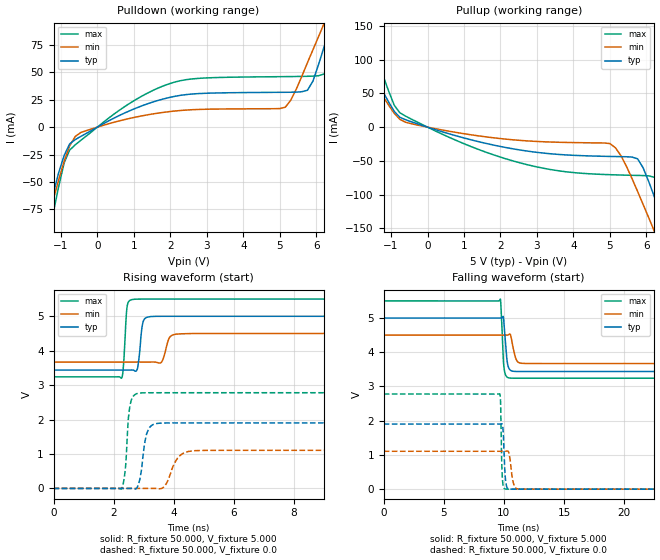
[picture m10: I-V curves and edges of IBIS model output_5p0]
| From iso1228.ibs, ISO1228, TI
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|   Model output_5p0
[Model] output_5p0
Model_type Output
Polarity   Non-Inverting
Enable   Active-High
Vmeas = 2.5
Vref = 0
Cref = 15pF
Rref = 1000
C_comp   0.978pF   1.050pF   0.889pF
[Temperature Range]   27.000   0.150k   -40.000
[Voltage Range]   5.000V   4.500V   5.500V
[Pullup Reference]   5.000V   4.500V   5.500V
[Pulldown Reference]   0.0V   0.0V   0.0V
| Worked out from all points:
|   slope of the pulldown table from 0 to 0.75 V, typ, clamps not added: 58.1 ohm
|   slope of the pullup table from 0 to 0.75 V, typ, clamps not added: 60.7 ohm
|   rising waveform, R_fixture 50.000, V_fixture 5.000: 20-80 % time 106ps typ, 156ps min, 85.7ps max; typ from 3.44 V to 5 V
|   rising waveform, R_fixture 50.000, V_fixture 0.0: 20-80 % time 187ps typ, 332ps min, 126ps max; typ from 0 V to 1.9 V
|   falling waveform, R_fixture 50.000, V_fixture 5.000: 20-80 % time 225ps typ, 313ps min, 176ps max; typ from 5 V to 3.44 V
|   falling waveform, R_fixture 50.000, V_fixture 0.0: 20-80 % time 143ps typ, 258ps min, 98.5ps max; typ from 1.9 V to 0 V
[Pulldown]
|Voltage   I(typ)   I(min)   I(max)
-5V       -815.5mA   -672.8mA   -1.202A
-1.515V   -105.6mA   -105.1mA   -136.1mA
-1.212V   -61.35mA   -66.74mA   -79.03mA
-909mV    -25.88mA   -31.11mA   -32.53mA
-606mV    -11.4mA    -8.566mA   -16.16mA
1.212V    19.31mA    10.22mA    28.12mA
5.152V    31.78mA    18.16mA    46.05mA
5.758V    33.62mA    58.73mA    46.36mA
6.212V    72.89mA    94.39mA    48.42mA
6.364V    89.22mA    106.5mA    53.15mA
6.667V    121.6mA    131.9mA    95.16mA
10V       660.1mA    546.8mA    912.1mA
[Pullup]
|Voltage   I(typ)   I(min)   I(max)
-5V       644mA      477.1mA    1.049A
-2.424V   204.2mA    153.2mA    323.8mA
-2.121V   160.1mA    122.2mA    245mA
-1.667V   102.5mA    83.45mA    148.2mA
-758mV    14.58mA    11.61mA    21.29mA
2.273V    -31.52mA   -18.45mA   -49.05mA
5V        -43.5mA    -24.42mA   -70.59mA
5.758V    -47.03mA   -95.47mA   -71.69mA
6.212V    -102.6mA   -154mA     -74.33mA
6.515V    -148.3mA   -193.8mA   -102.8mA
6.818V    -195mA     -237.4mA   -163.6mA
10V       -864.2mA   -796.2mA   -1.115A
[Ramp]
| variable   typ   min   max
dV/dt_r   1.142/0.185n   0.664/0.334n   1.668/0.127n
dV/dt_f   0.938/0.225n   0.498/0.317n   1.355/0.180n
R_load = 50.000
[Rising Waveform]
R_fixture= 50.000
V_fixture= 5.000
V_fixture_min= 4.500
V_fixture_max= 5.500
|time   V(typ)   V(min)   V(max)
0s        3.437V     3.67V      3.241V
2.27ns    3.437V     3.67V      3.207V
2.33ns    3.437V     3.67V      3.564V
2.46ns    3.437V     3.67V      5.319V
2.77ns    3.424V     3.67V      5.497V
3ns       4.873V     3.67V      5.5V
3.41ns    4.998V     3.667V     5.5V
3.9ns     5V         4.418V     5.5V
4.59ns    5V         4.498V     5.5V
100ns     5V         4.5V       5.5V
[Rising Waveform]
R_fixture= 50.000
V_fixture= 0.0
V_fixture_min= 0.0
V_fixture_max= 0.0
|time   V(typ)   V(min)   V(max)
0s        3.3nV      128.9nV    17.73nV
2.26ns    196.7nV    128.7nV    -19.15mV
2.39ns    -18.56uV   121nV      532.8mV
2.58ns    735.9uV    268.2nV    2.53V
2.81ns    70.08mV    1.698uV    2.76V
3.01ns    1.145V     -25.22uV   2.777V
3.31ns    1.852V     727.1uV    2.779V
4.27ns    1.902V     992.9mV    2.779V
5.12ns    1.902V     1.106V     2.779V
100ns     1.903V     1.107V     2.779V
[Falling Waveform]
R_fixture= 50.000
V_fixture= 5.000
V_fixture_min= 4.500
V_fixture_max= 5.500
|time   V(typ)   V(min)   V(max)
0s        5V         4.5V       5.5V
9.7ns     4.999V     4.5V       5.553V
9.77ns    4.998V     4.5V       5.209V
9.94ns    5.043V     4.5V       3.858V
10.03ns   4.711V     4.5V       3.488V
10.27ns   3.722V     4.499V     3.271V
10.56ns   3.47V      4.491V     3.244V
11.08ns   3.438V     3.747V     3.241V
11.86ns   3.437V     3.67V      3.241V
100ns     3.437V     3.67V      3.241V
[Falling Waveform]
R_fixture= 50.000
V_fixture= 0.0
V_fixture_min= 0.0
V_fixture_max= 0.0
|time   V(typ)   V(min)   V(max)
0s        1.903V     1.107V     2.779V
9.63ns    1.902V     1.107V     2.787V
9.72ns    1.902V     1.107V     2.524V
9.81ns    1.91V      1.107V     869.6mV
9.86ns    1.896V     1.107V     368.3mV
10.19ns   137.1mV    1.109V     2.71mV
10.41ns   8.114mV    1.06V      737.3uV
10.82ns   513.3uV    133.1mV    190.8uV
11.32ns   143.7uV    3.033mV    43.61uV
100ns     62.99nV    170.1nV    61.69nV
